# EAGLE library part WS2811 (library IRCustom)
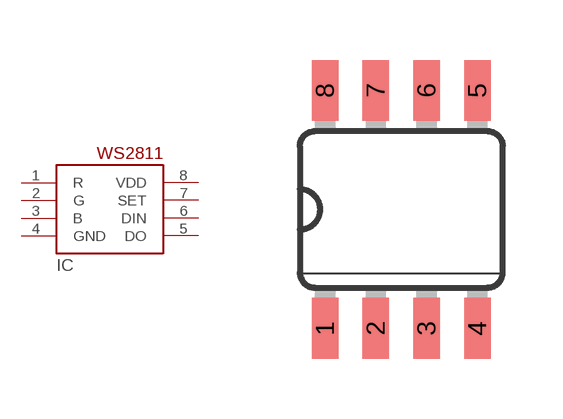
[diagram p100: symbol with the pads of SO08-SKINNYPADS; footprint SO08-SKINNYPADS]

Designator prefix IC

## WS2811-SOP8  [SO08-SKINNYPADS]
1  R  oc
2  G  oc
3  B  oc
4  GND  pwr
5  DO  out
6  DIN  in
7  SET  in
8  VDD  pwr

## Footprint SO08-SKINNYPADS (pad centres in mm)
smd 0.66 x 1.524: 1 -1.905,-2.973; 2 -0.635,-2.973; 3 0.635,-2.973; 4 1.905,-2.973; 5 1.905,2.973; 6 0.635,2.973; 7 -0.635,2.973; 8 -1.905,2.973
